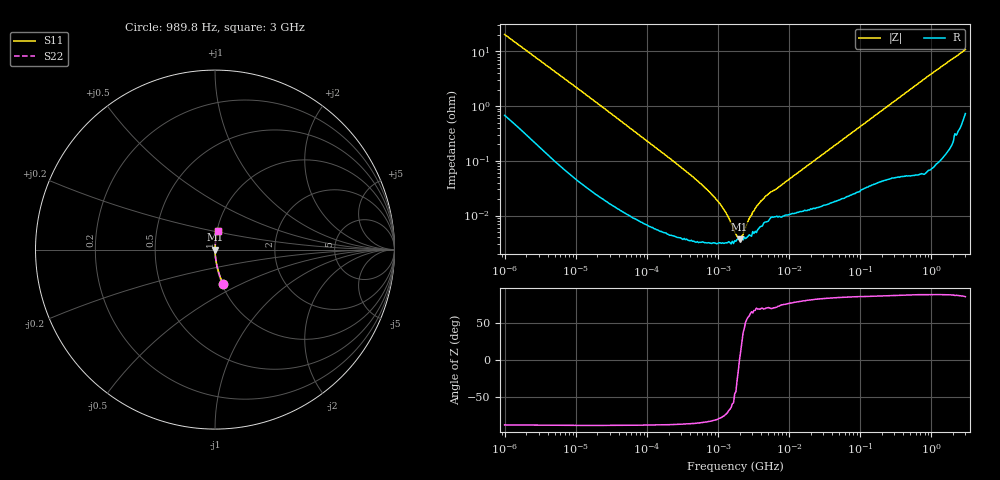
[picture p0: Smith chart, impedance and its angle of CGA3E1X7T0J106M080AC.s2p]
! S-Parameter Data Generated by TDK Corporation
! Copyright(C) 2022 TDK Corporation.
! All Rights Reserved.
! TDK P/N: CGA3E1X7T0J106M080AC (Multilayer Ceramic Chip Capacitor)
! Property: C=10uF
! Size(LxWxT): 1.6x0.8x0.8mm
! Model Type: s2p (Touchstone File Format Version 1.0)
! Frequency: DC=Yes Start=0.000989846400768MHz Stop=3000MHz 467points Log-sweep
! Model Generated on Feb. 7, 2022
! Port Assignments:
!  1 ---| |--- 2
! Applicable Conditions:
!  Temperature = 25 degC
!  DC Bias Voltage = 0 V
!  Small Signal Operation
! Terms and conditions regarding TDK Simulation Models
! (1)This simulation model is being provided solely for informational purposes. Please refer to the specifications of the products in terms of detailed characteristics of such products.
! (2)In no event shall TDK Corporation of any of its subsidiaries be liable for any loss or damage arising, directly or indirectly,
!  From any information contained in this simulation model, including, but not limited to loss or damages arising from any inaccuracies, omissions or errors in connection with such information.
! (3)Any and all copyrights on this simulation model are owned by TDK Corporation.
!  Duplication or redistribution of this simulation model without prior written permission from TDK Corporation is prohibited.
! (4)This simulation model is subject to any modification or change without any prior notice.
! (5)Neither TDK Corporation nor any of its subsidiaries shall make any warranty, express or implied,
!  Including but not limited to the correctness, implied warranties of merchantability and fitness for a particular purpose with respect to this simulation models.
! (6)The use of this simulation model shall be deemed to have consented to the terms and conditions hereof.
# Hz S MA R 50
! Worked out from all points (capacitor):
!   466 points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, 989.8 Hz to 3 GHz, reference 50 ohm
!   read as one part in series: C = 7.76 uF near 1.07 kHz
!   lowest |Z| = 3.66 mohm at 1.995 MHz (marker M1)
!   series resonance near 1.991 MHz, so ESL is about 820 pH
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989.8464  0.1993 -76.6  0.9733 11.5  0.9733 11.5  0.1993 -76.6
1709.24  0.1203 -81.4  0.9892 6.9  0.9892 6.9  0.1203 -81.4
2838.527  0.07466 -84.2  0.9953 4.3  0.9953 4.3  0.07466 -84.2
12024.64  0.01862 -87.8  0.9994 1.1  0.9994 1.1  0.01862 -87.8
146075.1  0.001587 -88.0  0.9999 0.1  0.9999 0.1  0.001587 -88.0
358360.3  0.0006373 -86.6  1 0.0  1 0.0  0.0006373 -86.6
643428.9  0.0003297 -84.4  1 0.0  1 0.0  0.0003297 -84.4
914132.1  0.0002067 -81.3  1 0.0  1 0.0  0.0002067 -81.3
1350401  0.0001001 -71.5  1 0.0  1 0.0  0.0001001 -71.5
1460002  8.21e-05 -66.9  1 0.0  1 0.0  8.21e-05 -66.9
1774518  4.611e-05 -42.7  1 0.0  1 0.0  4.611e-05 -42.7
1994879  3.659e-05 0.7  1 -0.0  1 -0.0  3.659e-05 0.7
2725709  8.821e-05 59.7  1 -0.0  1 -0.0  8.821e-05 59.7
2834164  9.603e-05 63.2  1 -0.0  1 -0.0  9.603e-05 63.2
3064190  0.0001162 63.9  0.9999 -0.0  0.9999 -0.0  0.0001162 63.9
3724282  0.000165 69.5  0.9999 -0.0  0.9999 -0.0  0.000165 69.5
4893958  0.0002364 70.9  0.9999 -0.0  0.9999 -0.0  0.0002364 70.9
6952943  0.0003245 73.1  0.9999 -0.0  0.9999 -0.0  0.0003245 73.1
2.073191e7  0.0009343 81.9  0.9999 -0.1  0.9999 -0.1  0.0009343 81.9
2.507343e8  0.01031 86.8  0.9995 -0.6  0.9995 -0.6  0.01031 86.8
1.038491e9  0.04063 86.6  0.9984 -2.3  0.9984 -2.3  0.04063 86.6
3e9  0.1069 80.0  0.9871 -6.1  0.9871 -6.1  0.1069 80.0
